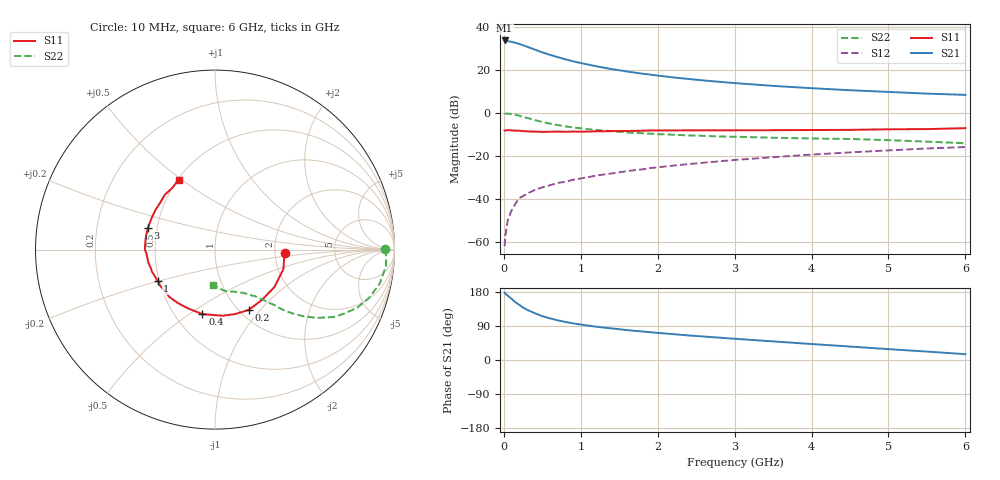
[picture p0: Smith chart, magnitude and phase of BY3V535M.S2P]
! SIEMENS Small Signal Semiconductors
! BFY420
! Si NPN RF SIEGET Grounded Emitter Transistor in MICRO-X
! VCE = 3.5 V  IC = 35 mA
! Common Emitter S-Parameters:  October  1996
# GHz  S  MA  R  50
!  f  S11  S21  S12  S22
! GHz  MAG  ANG  MAG  ANG  MAG  ANG  MAG  ANG
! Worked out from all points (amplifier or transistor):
!   36 points, 10 MHz to 6 GHz, reference 50 ohm
!   highest |S21| = 33.6 dB at 10 MHz (marker M1)
!   |S21| within 3 dB of that: start of sweep to 308.9 MHz
!   unconditionally stable (mu >= 1): 1.599 GHz to end of sweep
!   at 250 MHz: K = 0.39, MSG = 35.0 dB, |S12| = -38.6 dB
!   at 1.4 GHz: K = 0.98, MSG = 24.2 dB, |S12| = -28.2 dB
!   at 6 GHz: K = 1.05, MAG = 10.7 dB, |S12| = -15.9 dB
!   S11 on the Smith chart (normalised r, x): 10 MHz: 2.28, -0.11; 200 MHz: 1.10, -0.87; 400 MHz: 0.68, -0.56; 1 GHz: 0.49, -0.20; 3 GHz: 0.45, +0.13; 6 GHz: 0.50, +0.49
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0.01  0.3911 -2.9  47.86 177.9  0.0008 124.8  0.9451 0.1
0.02  0.3881 -7.2  47.49 174.9  0.0014 98.5  0.953 -1.3
0.05  0.3963 -15.8  46.01 169.9  0.0031 80.8  0.958 -5.4
0.1  0.3914 -32.2  44.61 161.6  0.0054 76.8  0.9364 -11.8
0.15  0.3836 -47.0  42.23 152.4  0.0077 73.3  0.8993 -17.4
0.2  0.3851 -60.8  39.83 145.5  0.0104 72.9  0.8574 -22.1
0.25  0.3761 -72.8  36.99 138.5  0.0117 67.4  0.8066 -26.1
0.3  0.371 -83.5  34.34 132.7  0.0132 66.8  0.7626 -29.5
0.4  0.3661 -101.0  29.49 123.7  0.0161 65.0  0.679 -34.1
0.5  0.3604 -114.9  25.29 115.6  0.0185 63.5  0.6123 -37.2
0.6  0.3627 -125.3  22.18 109.9  0.0208 63.1  0.5604 -39.4
0.7  0.3665 -134.2  19.63 104.7  0.0235 63.0  0.519 -41.1
0.8  0.3623 -141.5  17.46 100.4  0.0251 62.4  0.4848 -42.2
1  0.3646 -151.4  14.31 93.5  0.0299 64.8  0.4362 -43.8
1.1  0.3664 -156.1  13.15 90.6  0.0321 64.5  0.4165 -45.0
1.6  0.3793 -172.4  9.101 78.9  0.0443 64.0  0.3506 -48.7
2.2  0.3901 174.8  6.637 68.2  0.0594 62.1  0.3101 -53.5
3  0.3927 161.8  4.902 56.1  0.0803 57.2  0.2786 -59.6
3.5  0.3945 153.5  4.219 49.1  0.0933 53.9  0.2637 -63.5
4.5  0.4016 139.5  3.342 35.5  0.1203 45.4  0.2469 -72.1
5.5  0.4185 124.3  2.791 22.2  0.1483 36.3  0.214 -84.4
6  0.4397 117.4  2.609 15.4  0.1608 31.3  0.1965 -92.5
